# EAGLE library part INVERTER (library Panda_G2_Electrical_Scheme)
Inverter
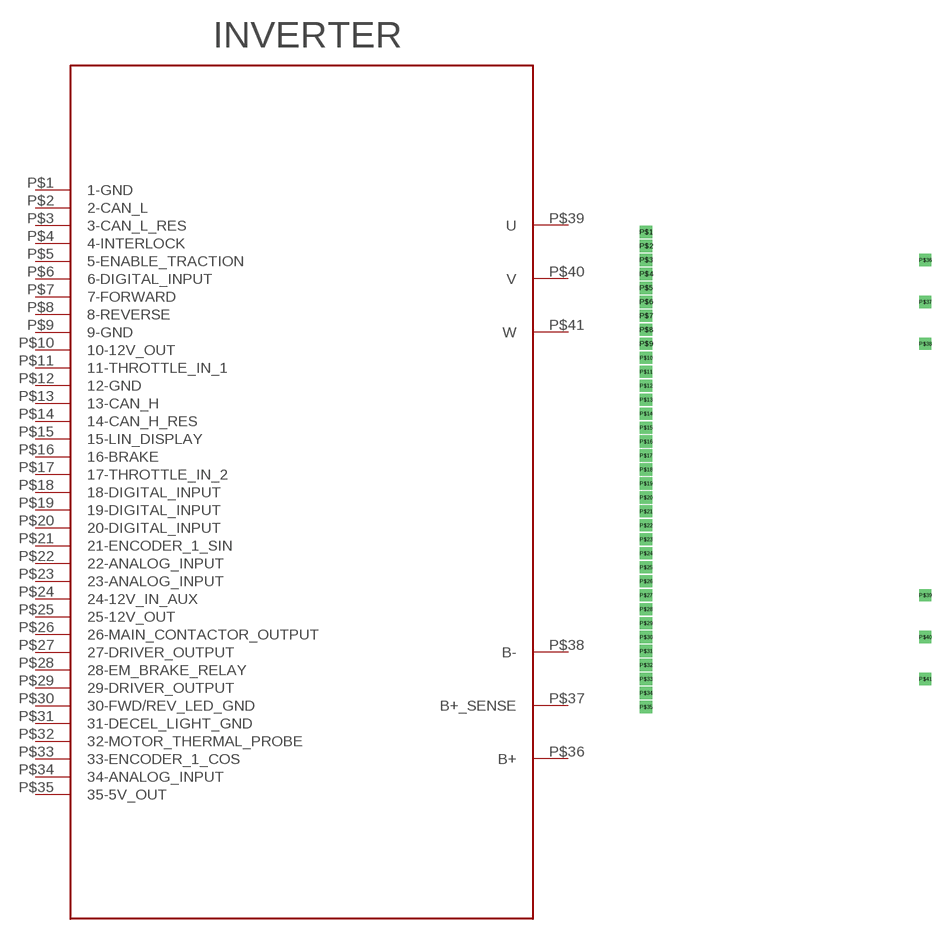
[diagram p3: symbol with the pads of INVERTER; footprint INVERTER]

Designator prefix -

## INVERTER  [INVERTER]
P$1  1-GND
P$2  2-CAN_L
P$3  3-CAN_L_RES
P$4  4-INTERLOCK
P$5  5-ENABLE_TRACTION
P$6  6-DIGITAL_INPUT
P$7  7-FORWARD
P$8  8-REVERSE
P$9  9-GND
P$10  10-12V_OUT
P$11  11-THROTTLE_IN_1
P$12  12-GND
P$13  13-CAN_H
P$14  14-CAN_H_RES
P$15  15-LIN_DISPLAY
P$16  16-BRAKE
P$17  17-THROTTLE_IN_2
P$18  18-DIGITAL_INPUT
P$19  19-DIGITAL_INPUT
P$20  20-DIGITAL_INPUT
P$21  21-ENCODER_1_SIN
P$22  22-ANALOG_INPUT
P$23  23-ANALOG_INPUT
P$24  24-12V_IN_AUX
P$25  25-12V_OUT
P$26  26-MAIN_CONTACTOR_OUTPUT
P$27  27-DRIVER_OUTPUT
P$28  28-EM_BRAKE_RELAY
P$29  29-DRIVER_OUTPUT
P$30  30-FWD/REV_LED_GND
P$31  31-DECEL_LIGHT_GND
P$32  32-MOTOR_THERMAL_PROBE
P$33  33-ENCODER_1_COS
P$34  34-ANALOG_INPUT
P$35  35-5V_OUT
P$36  B+
P$37  B+_SENSE
P$38  B-
P$39  U
P$40  V
P$41  W

## Footprint INVERTER (pad centres in mm)
drill 0.6 square: P$1 -6.35,54.61; P$2 -6.35,53.34; P$3 -6.35,52.07; P$4 -6.35,50.8; P$5 -6.35,49.53; P$6 -6.35,48.26; P$7 -6.35,46.99; P$8 -6.35,45.72; P$9 -6.35,44.45; P$10 -6.35,43.18; P$11 -6.35,41.91; P$12 -6.35,40.64; P$13 -6.35,39.37; P$14 -6.35,38.1; P$15 -6.35,36.83; P$16 -6.35,35.56; P$17 -6.35,34.29; P$18 -6.35,33.02; P$19 -6.35,31.75; P$20 -6.35,30.48; P$21 -6.35,29.21; P$22 -6.35,27.94; P$23 -6.35,26.67; P$24 -6.35,25.4; P$25 -6.35,24.13; P$26 -6.35,22.86; P$27 -6.35,21.59; P$28 -6.35,20.32; P$29 -6.35,19.05; P$30 -6.35,17.78; P$31 -6.35,16.51; P$32 -6.35,15.24; P$33 -6.35,13.97; P$34 -6.35,12.7; P$35 -6.35,11.43; P$36 19.05,52.07; P$37 19.05,48.26; P$38 19.05,44.45; P$39 19.05,21.59; P$40 19.05,17.78; P$41 19.05,13.97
